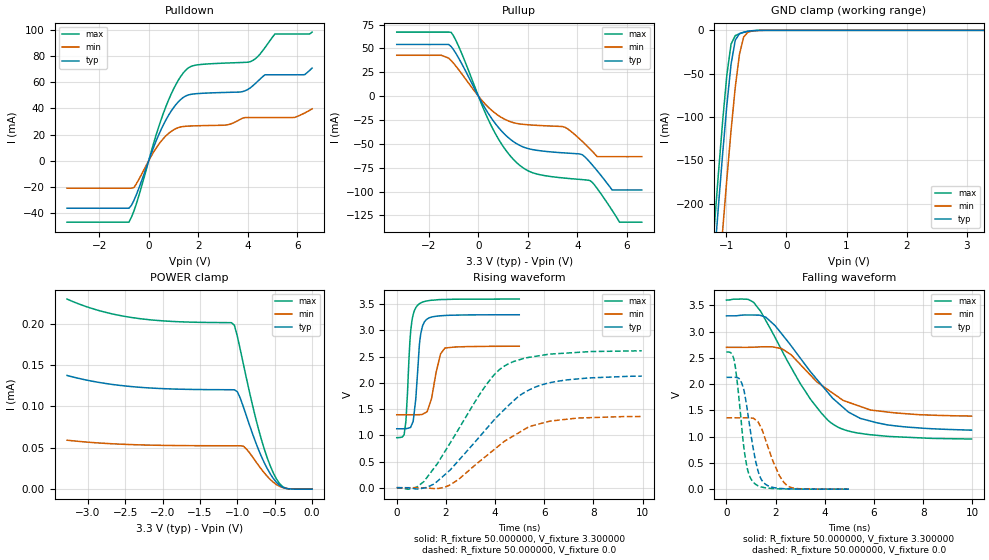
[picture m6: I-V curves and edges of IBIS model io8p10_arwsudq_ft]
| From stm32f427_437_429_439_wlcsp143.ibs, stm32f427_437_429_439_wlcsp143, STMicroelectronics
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|   Model io8p10_arwsudq_ft
[Model]  io8p10_arwsudq_ft
Model_type I/O
Polarity   Non-Inverting
Enable   Active-Low
Vinl =   0.990000V
Vinh =   2.310000V
Vmeas =  1.650000V
Cref =   40.000000pF
Rref =   100.000000M
Vref =   0.0V
C_comp   2.905500pF   2.826300pF   2.987900pF
[Temperature Range]   25.000000   0.125000k   -40.000000
[Pullup Reference]   3.300000V   2.700000V   3.600000V
[Pulldown Reference]   0.0V   0.0V   0.0V
[POWER Clamp Reference]   3.300000V   2.700000V   3.600000V
[GND Clamp Reference]   0.0V   0.0V   0.0V
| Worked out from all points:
|   slope of the pulldown table from 0 to 0.495 V, typ, clamps not added: 20.9 ohm
|   slope of the pullup table from 0 to 0.495 V, typ, clamps not added: 22.6 ohm
|   GND clamp passes 1 mA (typ) near -0.62 V on its own axis
|   rising waveform, R_fixture 50.000000, V_fixture 3.300000: 20-80 % time 215ps typ, 342ps min, 189ps max; typ from 1.12 V to 3.3 V
|   rising waveform, R_fixture 50.000000, V_fixture 0.0: 20-80 % time 2.52ns typ, 2.31ns min, 2.11ns max; typ from 0 V to 2.13 V
|   falling waveform, R_fixture 50.000000, V_fixture 3.300000: 20-80 % time 2.33ns typ, 2.09ns min, 2.04ns max; typ from 3.3 V to 1.12 V
|   falling waveform, R_fixture 50.000000, V_fixture 0.0: 20-80 % time 461ps typ, 655ps min, 370ps max; typ from 2.13 V to 0 V
[Pulldown]
|Voltage   I(typ)   I(min)   I(max)
-3.3V     -36.4mA    -21.08mA   -47.09mA
-800mV    -36.4mA    -21.08mA   -47.09mA
-600mV    -30.5mA    -20.54mA   -38.69mA
700mV     31.4mA     19.11mA    41.71mA
1.2V      45.15mA    25.37mA    61.75mA
1.6V      50.35mA    26.5mA     71.06mA
3.1V      52.28mA    27.26mA    74.76mA
4.1V      55.71mA    33.04mA    75.8mA
4.7V      65.81mA    33.04mA    86.69mA
5.1V      65.81mA    33.04mA    97.04mA
6.3V      65.87mA    36.5mA     97.04mA
6.6V      70.93mA    39.72mA    98.49mA
[Pullup]
|Voltage   I(typ)   I(min)   I(max)
-3.3V     54.25mA    42.91mA    67.2mA
-1.1V     52mA       37.31mA    66.91mA
500mV     -22.07mA   -14mA      -30.03mA
1.5V      -49.1mA    -28.3mA    -68.56mA
2.2V      -56.05mA   -30.32mA   -80.35mA
3.5V      -59.53mA   -32.66mA   -85.92mA
4.2V      -61.44mA   -47.49mA   -87.46mA
4.5V      -69.08mA   -55.13mA   -88.39mA
4.8V      -78.24mA   -63.4mA    -96.88mA
5.4V      -98.3mA    -63.4mA    -119.6mA
5.7V      -98.3mA    -63.4mA    -132.1mA
6.6V      -98.3mA    -63.4mA    -132.1mA
[GND_clamp]
|Voltage   I(typ)   I(min)   I(max)
-3.3V     -2.319A    -2.397A    -2.292A
-1.2V     -266mA     -356.2mA   -228.4mA
-1.13V    -203.2mA   -293mA     -165.3mA
-1.06V    -142.7mA   -231.3mA   -105.2mA
-990mV    -86.51mA   -171.7mA   -51.78mA
-920mV    -39.3mA    -115.7mA   -15.93mA
-850mV    -11.37mA   -65.76mA   -6.097mA
-780mV    -3.83mA    -27.55mA   -3.88mA
-710mV    -2.09mA    -7.747mA   -2.382mA
-640mV    -1.147mA   -2.129mA   -1.22mA
-570mV    -523.9uA   -800uA     -476.9uA
3.28V     0A         0A         0A
[POWER_clamp]
|Voltage   I(typ)   I(min)   I(max)
-3.28V    137.3uA    59.14uA    229.6uA
-2.36V    123.4uA    53.65uA    206.6uA
-1.08V    120.1uA    52.41uA    201.1uA
-1.04V    120uA      52.41uA    198uA
-1V       117.7uA    52.4uA     184.5uA
-920mV    99.46uA    51.91uA    151.2uA
-720mV    48.42uA    29.12uA    73.51uA
-600mV    24.82uA    15.47uA    37.72uA
-520mV    13.1uA     8.45uA     19.84uA
-440mV    5.058uA    3.61uA     7.276uA
-360mV    1.193uA    1.129uA    1.311uA
0V        0A         0A         0A
[Ramp]
| variable   typ   min   max
dV/dt_r  1.26708/2.51445n   0.81144/2.30948n   1.56461/2.11080n
dV/dt_f  1.28286/2.32002n   0.77634/2.07752n   1.57505/2.03651n
R_load = 50.000000
[Rising Waveform]
R_fixture= 50.000000
V_fixture= 3.300000
V_fixture_min= 2.700000
V_fixture_max= 3.600000
|time   V(typ)   V(min)   V(max)
0s        1.124V     1.392V     954.3mV
310.3ps   1.126V     1.392V     1.043V
380.4ps   1.128V     1.392V     1.331V
570.6ps   1.159V     1.392V     2.996V
670.7ps   1.272V     1.391V     3.306V
830.8ps   2.082V     1.392V     3.47V
981ps     2.944V     1.395V     3.527V
1.251ns   3.223V     1.469V     3.564V
1.962ns   3.285V     2.665V     3.591V
4.985ns   3.3V       2.7V       3.599V
[Rising Waveform]
R_fixture= 50.000000
V_fixture= 0.0
V_fixture_min= 0.0
V_fixture_max= 0.0
|time   V(typ)   V(min)   V(max)
0s        348.8uV    197.7uV    665.1uV
580.6ps   -7.684mV   200.6uV    -18.72mV
1.101ns   -5.304mV   -2.568mV   115.4mV
1.522ns   70.65mV    -16.65mV   376.5mV
2.142ns   324.6mV    46.06mV    829.7mV
3.664ns   1.132V     613.8mV    1.977V
4.505ns   1.55V      921mV      2.354V
5.285ns   1.842V     1.138V     2.48V
6.186ns   1.998V     1.264V     2.547V
9.97ns    2.129V     1.359V     2.612V
[Falling Waveform]
R_fixture= 50.000000
V_fixture= 3.300000
V_fixture_min= 2.700000
V_fixture_max= 3.600000
|time   V(typ)   V(min)   V(max)
0s        3.3V       2.7V       3.599V
900.9ps   3.315V     2.7V       3.609V
1.101ns   3.315V     2.702V     3.559V
1.602ns   3.273V     2.711V     3.209V
2.262ns   2.948V     2.671V     2.634V
3.423ns   2.233V     2.167V     1.71V
4.444ns   1.681V     1.789V     1.205V
4.965ns   1.467V     1.654V     1.107V
6.086ns   1.268V     1.494V     1.027V
9.97ns    1.124V     1.392V     954.3mV
[Falling Waveform]
R_fixture= 50.000000
V_fixture= 0.0
V_fixture_min= 0.0
V_fixture_max= 0.0
|time   V(typ)   V(min)   V(max)
0s        2.129V     1.359V     2.612V
300.3ps   2.13V      1.359V     2.483V
460.5ps   2.118V     1.358V     1.953V
620.6ps   2.022V     1.358V     1.192V
860.9ps   1.469V     1.36V      370.2mV
1.091ns   771mV      1.35V      133.6mV
1.481ns   142.1mV    1.09V      35.66mV
2.152ns   15.87mV    257.7mV    6.465mV
2.452ns   7.311mV    76.29mV    4.562mV
4.985ns   348.8uV    197.7uV    665.1uV
